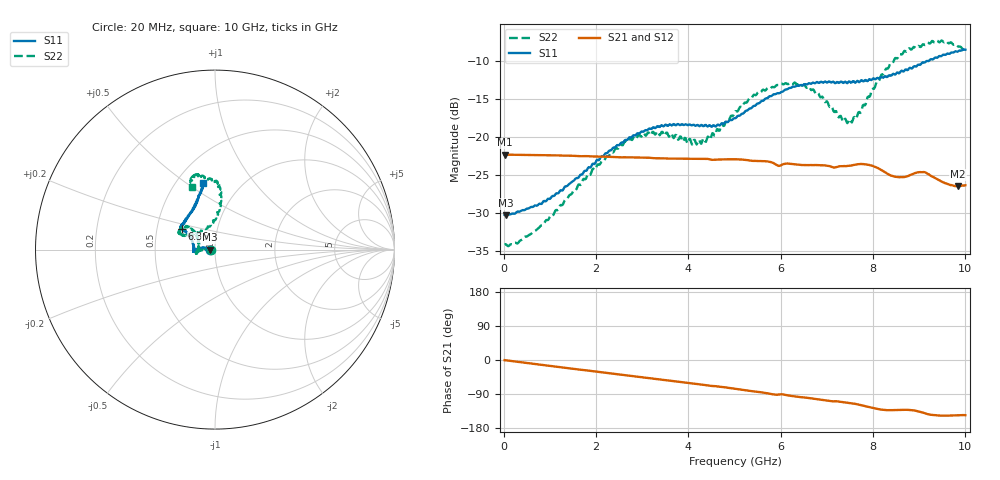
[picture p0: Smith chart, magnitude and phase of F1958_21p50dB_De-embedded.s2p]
! Integrated Device Technology
! Corporate Headquarters
! 6024 Silver Creek Valley Road
! San Jose, CA 95138  USA
! Phone:  1-408-284-8200
! Toll Free:  1-800-223-1366
! Webpage:  http://www.idt.com/
! Timing and RF Division
! 515 Groton Road, Suite 102
! Westford, MA 01886-6024
! Device:  F1958
! Description: 7-bit 0.25 dB Digital Step Attenuator
! Frequency:  0.001 -  6.000 GHz
! Package:  4x4 mm Thin QFN Plastic Package: 24 pin
! Ports:  2 RF, 12 DC
!  Pin  1  = D0
!  Pin  2  = VDD
!  Pin  3  = VMODE
!  Pin  4  = GND
!  Pin  5  = RF1  =  Port 1
!  Pin  6  = GND
!  Pin  7  = GND
!  Pin  8  = GND
!  Pin  9  = GND
!  Pin 10  = GND
!  Pin 11  = GND
!  Pin 12  = GND
!  Pin 13  = GND
!  Pin 14  = RF2  =  Port 2
!  Pin 15  = GND
!  Pin 16  = LE
!  Pin 17  = CLK
!  Pin 18  = DATA
!  Pin 19  = D6
!  Pin 20  = D5
!  Pin 21  = D4
!  Pin 22  = D3
!  Pin 23  = D2
!  Pin 24  = D1
! State:  86
! Atten State:  21.50 dB
! Voltage:  +3.30 Volts
! Current:  0.258 mA
! Data:  The device was measured on a F1958 evaluation board which has
!  individual transmission lines to the RF pins.  Data was collected
!  using a calibrated network analyzer.  The evaluation board was
!  de-embedded using Automatic Fixture Removal (AFR).
!  The reference plane is the edge of the package pin.
! Misc:
!  Action Tracker AT0419
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# GHz S dB R 50
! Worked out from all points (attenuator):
!   500 points, 20 MHz to 10 GHz, reference 50 ohm
!   highest |S21| = -22.33 dB at 20 MHz (marker M1); lowest = -26.5 dB at 9.84 GHz (marker M2)
!   lowest |S11| = -30.3 dB at 40 MHz (marker M3), VSWR 1.06, Z = 47 - j0.0428 ohm
!   |S11| at or under -10 dB: start of sweep to 9.158 GHz; 9.18555 GHz to 9.201076 GHz (15.53 MHz wide, 0.169 % of centre)
!   |S22| runs from -34.4 to -7.3 dB; largest |S21 - S12| = 0.00034
!   S11 on the Smith chart (normalised r, x): 20 MHz: 0.94, -0.00; 6.36 GHz: 0.67, +0.16; 10 GHz: 0.67, +0.58
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0.02  -30.29 -178.9  -22.33 -0.4  -22.33 -0.3  -34.19 -177.8
0.04  -30.33 -179.1  -22.34 -0.7  -22.33 -0.6  -34.13 -176.9
0.72  -29.06 172.5  -22.40 -11.2  -22.39 -11.2  -32.20 -180.0
1.7  -24.95 171.0  -22.54 -26.0  -22.53 -26.0  -25.89 179.3
2.6  -20.65 176.9  -22.68 -39.6  -22.66 -39.6  -20.86 -176.1
3.36  -18.67 -175.5  -22.82 -51.2  -22.82 -51.3  -19.60 -168.0
4.26  -18.51 -179.7  -22.88 -64.4  -22.90 -64.5  -20.76 169.4
4.52  -18.59 174.3  -23.02 -68.5  -23.03 -68.6  -19.51 154.5
5.02  -17.53 161.0  -22.94 -76.0  -22.96 -76.0  -16.61 139.8
5.58  -15.27 150.7  -23.19 -85.3  -23.21 -85.3  -14.04 140.1
6.36  -13.24 148.3  -23.65 -97.0  -23.66 -96.9  -13.15 153.7
6.68  -12.90 146.9  -23.72 -101.4  -23.72 -101.3  -13.80 155.0
7.32  -12.72 141.7  -23.87 -110.9  -23.87 -110.8  -17.54 134.9
7.5  -12.73 138.6  -23.80 -113.5  -23.80 -113.4  -17.69 116.8
7.68  -12.69 135.8  -23.59 -117.4  -23.59 -117.3  -16.77 99.1
7.9  -12.51 129.4  -23.67 -123.8  -23.66 -123.8  -14.68 89.3
8.34  -11.89 119.5  -24.94 -132.5  -24.95 -132.6  -10.82 83.2
8.68  -11.26 112.8  -25.28 -131.5  -25.27 -131.4  -8.66 87.6
9.04  -10.39 107.4  -24.65 -137.6  -24.65 -137.6  -8.11 95.3
9.26  -9.75 105.2  -25.16 -144.4  -25.17 -144.5  -7.49 100.3
9.84  -8.73 100.4  -26.50 -145.9  -26.52 -145.7  -8.08 109.8
10  -8.51 100.2  -26.37 -145.6  -26.40 -145.5  -8.61 110.3
